[IBIS ver]	1.1
[File name]  	mpc555m.ibs
[File Rev]	0.3
[Date]   Tuesday,04/Dec/2001
[Source]	File originated at Oakhill
[Notes]		Model created by Sukanya Rajagopal(edit rd)
[Disclaimer]	This information is for modeling purposes only
|		and is not guarenteed.
|   This applies to revisions M and later
|   CLKOUT and ECKBUCK output drive changed
|   CLKOUT now 30/90
|   ECKBUCK now 25/50
|   Modified for fast [test] mode vs Normal [slow] comments
|   to agree with reference manual
[Component]	MPC555
[Manufacturer]  Motorola
| Package type  PBGA
[Package]
R_pkg   21.0m   7.00m   36m
L_pkg   3.42nH   0.71nH   6.12nH
C_pkg   0.81pf   0.55pf   1.06pf
[Pin]	  signal_name	model_name	R_pin   L_pin  C_pin
|   mohm   nh   pf
|   POWER AND GROUND PINS
A1	  VDDH		POWER		23	3.81	1.01
A7	  VRL		POWER		25	3.76	0.71
A16	  VDDH		POWER		28	4.13	0.77
A20	  VDDH		POWER		22	3.68	0.97
B2	  VDDH		POWER		23	3.81	1.01
B7	  VRH		POWER		15	2.45	0.72
B19	  VDDH		POWER		22	3.68	0.97
C7	  VDDA		POWER		11	1.77	0.71
D6   VDDI   POWER
D16   VDDI   POWER
D17   VDDL   POWER
E4   VDDL   POWER
J4   VDDSRAM   POWER		8	1.09	0.7
K4   VDDL   POWER
K17   VDDL   POWER
P17   VPP   POWER		19	2.54	0.81
P20   VDDH		POWER   25	3.91	0.72
R17   VDDL   POWER
R18   VDDF		POWER   28	3.9	0.83
R19   XFC		POWER   21	3.06	0.74
R20	  VDDSYN	POWER   27	3.94	0.74
T4   VDDL   POWER
T17   VDDI   POWER
T18	  KAPWR		POWER   19	3.07	0.83
T20	  EXTAL		POWER   27	4.32	0.85
U5   VDDI   POWER
U10   VDDL   POWER
U15   VDDL   POWER
W2	  VDDH		POWER   27	4.11	1.06
W19	  VDDH		POWER   26	4.04	1.03
Y1	  VDDH		POWER   27	4.11	1.06
Y20	  VDDH		POWER   26	4.04	1.03
D7	  VSSA		GND		9	1.27	0.74
P19	  VSSF		GND   15	2.37	0.74
T19	  VSSSYN	GND   22	3.46	0.77
U20	  XTAL		POWER   32	4.76	0.85
|   INPUT ONLY PINS
H3	  CNRX0 	in_5v   26	3.32	0.79
J1	  TCKDXCK	in_3v   23	3.51	0.68
J3	  TRSTB   in_3v   12	1.6	0.69
K1	  TMS		in_3v   23	3.49	0.68
K2	  TDIDSDI	in_3v   17	2.46	0.67
K20	  ACNRX0	in_5v   24	3.58	0.69
M19	  ECK		in_5v   12	2.01	0.71
N17	  RXD1QGP1	in_5v   9	1.29	0.73
N19	  RXD2GP1	in_5v   13	2.12	0.7
P18	  EPEE		in_5v   25	3.34	0.81
U18	  EXTCLK	in_extclk   18	2.93	0.87
V19	  PORESETB	in_3v   30	4.49	0.93
Y18	  IRQ6BMCK2	in_3v   29	4.41	0.8
Y19	  IRQ7BMCK3	in_3v   34	5.14	0.96
|  OUTPUT ONLY PINS
|  Pins in this section have the option of using full strength(50pf load)
|  or half strength(25pf load). The default for these pins use full
|  strength drivers(model : out_3vf). To select half strength drivers
|  (out_3vh), all of the pins in this section must be changed.
|  The models available are:
|  Full strength : out_3vf
|  Half strength : out_3vh
J2	  TDODSDO	out_3vf   18	2.69	0.69
P4	  CS0B		out_3vf   10	1.42	0.73
R2	  CS3B		out_3vf   19	2.96	0.73
R3	  CS2B		out_3vf   26	3.35	0.8
R4	  CS1B		out_3vf   21	3.11	0.81
T1	  OEB		out_3vf   28	4.28	0.75
L1	  IWPIVFLS1	out_3vf   23	3.69	0.69
L2	  IWPOVFLS 	out_3vf   17	2.58	0.68
U17	  RCFBTXP	out_3vf   13	1.89	0.95
|  OUTPUT ONLY PINS
|  Pins in this section have the option of using normal mode or fast [test] mode
|  and the slew rate in both the cases is 200ns.(slow slew rate).The default
|  for these pins operate in normal mode (model : out_5v_200). To select fast
|  [test] mode (out_5v_200tm), all of the pins in this section must be changed.
|  The models available are:
|  Normal mode : out_5v_200
|  fast [test] mode   : out_5v_200tm
H4	  BCNTX0   out_5v_200   17	1.98	0.78
K19	  ACNTX0	out_5v_200   17	2.58	0.69
N18	  TXD1QGP0 	out_5v_200   27	3.59	0.82
N20	  TXD2QGP0 	out_5v_200   20	3.24	0.7
|  OUTPUT ONLY CLOCK PINS
|  5v Eng. clk have the option of using full drive strength(50pf load)
|  or half drive strength(25pf load).The default for this pin uses full
|  strength driver(model : out_5vf_clk). To select half strength driver
|  (out_5vh_clk), the pin in this section must be changed.
|  This pin changed on revision M and later.
|  The models available are:
|  Full Strength : out_5vf_clk
|  Half Strength : out_5vh_clk
U19	  ECKBUCK	out_5vf_clk	 25	3.75	0.84
|  OUTPUT ONLY PINS
|  3v clkout pin have the option of using full drive strength(90pf load)
|  or half drive strength(30pf load).The default for this pin use full
|  strength driver(model : out_3vf_clk). To select half strength driver
|  (out_3vh_clk), the pin in this section must be changed.
|  This pin changed on revision M and later.
|  The models available are:
|  Full Strength : out_3vf_clk
|  Half Strength : out_3vh_clk
V18	  CLKOUT	out_3vf_clk	 23	3.63	0.92
|  I/O PINS(Address & Data) in this section have the option of using 3v
|  driver with full drive strength(50pf load) or half drive strength
|  (25pf load), or 5v driver with 200ns slew rate operating in normal or
|  fast [test] mode. The default is 3v driver with full drive strength
|  (io_35v_3vf).
|  To use other models,all the pins in this section need to be changed.
|  The Pullup and Pulldown data for these models contain both the driver and
|  clamp data. Seperate clamp data is also provided.
|  Available models are:
|   3v buffer with Full Drive strength  : io_35v_3vf
|   3v buffer with Half Drive strength  : io_35v_3vh
|   5v, 200ns slew rate buffer in Normal mode  : io_35v_5v_200
|   5v, 200ns slew rate buffer in fast [test] mode   : io_35v_5v_200tm
V6	  ADDRSGP8	io_35v_3vf   15	2.15	0.79
V5	  ADDRSGP9	io_35v_3vf   16	2.26	0.8
V4	  ADDRSGP10	io_35v_3vf   18	2.64	0.84
V3	  ADDRSGP11	io_35v_3vf   14	2.26	0.85
W1	  ADDRSGP12	io_35v_3vf   33	5.13	0.89
Y2	  ADDRSGP13	io_35v_3vf   33	5.06	0.89
W3	  ADDRSGP14	io_35v_3vf   25	3.8	0.86
Y3	  ADDRSGP15	io_35v_3vf   32	4.78	0.85
W4	  ADDRSGP16	io_35v_3vf   24	3.61	0.84
Y4	  ADDRSGP17	io_35v_3vf   30	4.56	0.82
W5	  ADDRSGP18	io_35v_3vf   21	3.17	0.78
Y5	  ADDRSGP19	io_35v_3vf   28	4.24	0.78
W6	  ADDRSGP20	io_35v_3vf   21	3.07	0.78
Y6	  ADDRSGP21	io_35v_3vf   27	4.08	0.76
V7	  ADDRSGP22	io_35v_3vf   15	2.09	0.75
W7	  ADDRSGP23	io_35v_3vf   20	2.96	0.75
Y7	  ADDRSGP24	io_35v_3vf   27	4.01	0.75
Y8	  ADDRSGP25	io_35v_3vf   26	3.78	0.73
W8	  ADDRSGP26	io_35v_3vf   19	2.81	0.74
V8	  ADDRSGP27	io_35v_3vf   13	1.83	0.74
U8	  ADDRSGP28	io_35v_3vf   8	1.07	0.76
U9	  ADDRSGP29	io_35v_3vf   7	0.82	0.74
U7	  ADDRSGP30	io_35v_3vf   9	1.21	0.78
U6	  ADDRSGP31	io_35v_3vf   8	1.27	0.79
U11	  DATASGP29	io_35v_3vf   7	0.91	0.7
U12	  DATASGP27   io_35v_3vf   8	1.06	0.7
U13	  DATASGP25	io_35v_3vf   9	1.31	0.71
U14	  DATASGP23   io_35v_3vf   9	1.38	0.73
U16	  DATASGP20	io_35v_3vf   13	2.11	0.81
V9	  DATASGP31	io_35v_3vf   13	1.83	0.74
V10	  DATASGP30   io_35v_3vf   12	1.57	0.7
V11	  DATASGP28	io_35v_3vf   11	1.52	0.69
V12	  DATASGP26	io_35v_3vf   11	1.58	0.69
V13	  DATASGP24	io_35v_3vf   12	1.77	0.7
V14	  DATASGP22	io_35v_3vf   12	1.76	0.71
V15   DATASGP21	io_35v_3vf   15	2.25	0.74
V16	  DATASGP19	io_35v_3vf   15	2.28	0.73
V17	  DATASGP18   io_35v_3vf   17	2.61	0.76
W9	  DATASGP1	io_35v_3vf   19	2.77	0.74
W10	  DATASGP3   io_35v_3vf   18	2.58	0.7
W11   DATASGP5   io_35v_3vf   18	2.54	0.7
W12	  DATASGP7	io_35v_3vf   18	2.53	0.69
W13	  DATASGP9   io_35v_3vf   18	2.68	0.71
W14	  DATASGP11   io_35v_3vf   19	2.7	0.72
W15   DATASGP13	io_35v_3vf   19	2.84	0.73
W16	  DATASGP15	io_35v_3vf   20	2.97	0.73
W17	  DATASGP17	io_35v_3vf   21	3.21	0.75
Y9	  DATASGP0	io_35v_3vf   25	3.72	0.72
Y10   DATASGP2	io_35v_3vf   24	3.52	0.69
Y11	  DATASGP4	io_35v_3vf   24	3.51	0.69
Y12	  DATASGP6   io_35v_3vf   24	3.56	0.69
Y13	  DATASGP8	io_35v_3vf   25	3.62	0.71
Y14	  DATASGP10   io_35v_3vf   25	3.69	0.71
Y15	  DATASGP12	io_35v_3vf   26	3.78	0.72
Y16	  DATASGP14	io_35v_3vf   26	3.93	0.74
Y17	  DATASGP16	io_35v_3vf   28	4.1	0.76
|   I/O PINS in this section use 3v supply with 50pf load. To have
|   half the drive strength(25pf load) all the pins in this section
|   need to be changed. Available models are:
|   3v buffer with Full Drive strength  : io_3vf
|   3v buffer with Half Drive strength  : io_3vh
R1	  RDWRB   io_3vf   26	3.84	0.73
T3	  TSIZ1		io_3vf   13	1.97	0.77
U1	  TSIZ0		io_3vf   29	4.55	0.79
U2	  TAB		io_3vf   23	3.33	0.78
U3	  TSB		io_3vf   17	2.75	0.8
U4	  BDIP		io_3vf   14	2.24	0.84
V1	  BURSTB	io_3vf   30	4.62	0.82
V2	  BIBSTSB	io_3vf   20	3.35	0.85
N1	  WEBAT0	io_3vf   24	3.52	0.68
P1	  WEBAT1	io_3vf   26	3.98	0.72
P2	  WEBAT2	io_3vf   20	3.07	0.72
P3	  WEBAT3	io_3vf   13	2.02	0.71
N2	  BRBLWP2	io_3vf   30	3.81	0.77
N3	  BGBLWP1   io_3vf   22	2.8	0.76
N4	  BB_BLWP3	io_3vf   19	2.54	0.78
| I/O PINS in this section use 5v supply with slew rate of 50ns.To have
| fast [test] mode all the pins in this section need to be changed.
| Available modes are:
| 5v fast buffer in normal operation   : io_5v_50
| 5v fast buffer in fast [test] mode operation : io_5v_50tm
L18	  PCS0QGP	io_5v_50   42	5.53	0.91
L17	  PCS1QGP	io_5v_50   41	4.14	0.95
M18	  PCS2QGP	io_5v_50   42	6.12	0.92
M17	  PCS3QGP	io_5v_50   22	2.99	0.87
L19	  MOSIQGP4 	io_5v_50   18	2.51	0.71
L20	  MOSIQGP5	io_5v_50   18	2.96	0.69
M20	  SCKQGP6	io_5v_50   24	3.61	0.69
|   I/O PINS in this section use 5v supply with 200ns slew and
|   operate in normal mode. To operate in fast [test] mode, all the pins
|   in this section need to be changed.
|   Available modes are:
|   5v slow buffer in normal operation   : io_5v_200
|   5v slow buffer in fast [test] mode operation : io_5v_200tm
D3	  ATPUO		io_5v_200   11	1.78	0.94
A2	  ATPU1		io_5v_200   29	4.66	0.96
D4	  ATPU2		io_5v_200   12	1.55	0.64
C3	  ATPU3		io_5v_200   15	2.51	0.86
A3	  ATPU4		io_5v_200   28	4.46	0.85
D5	  ATPU5		io_5v_200   13	1.59	0.64
B3	  ATPU6		io_5v_200   23	3.68	0.87
C4	  ATPU7		io_5v_200   19	2.83	0.84
A4	  ATPU8		io_5v_200   30	4.62	0.83
C5	  ATPU9		io_5v_200   17	2.35	0.72
B4	  ATPU10	io_5v_200   22	3.47	0.79
B5	  ATPU11	io_5v_200   16	2.59	0.74
A5	  ATPU12	io_5v_200   26	3.93	0.73
C6	  ATPU13	io_5v_200   13	1.9	0.6
B6	  ATPU14	io_5v_200   20	2.9	0.74
A6	  ATPU15	io_5v_200   21	3.37	0.71
C2	  AT2CLK	io_5v_200   25	3.85	0.89
H2	  BTPU0		io_5v_200   19	2.69	0.71
H1	  BTPU1		io_5v_200   25	3.83	0.72
G1	  BTPU2		io_5v_200   24	3.67	0.7
G2	  BTPU3		io_5v_200   35	4.65	0.84
G3	  BTPU4		io_5v_200   14	2	0.73
F1	  BTPU5		io_5v_200   26	3.87	0.72
F2	  BTPU6		io_5v_200   36	4.97	0.85
E1	  BTPU7		io_5v_200   29	4.53	0.77
F3	  BTPU8		io_5v_200   14	2.2	0.78
G4	  BTPU9		io_5v_200   10	1.08	0.79
E2	  BTPU10	io_5v_200   22	3.33	0.78
D1	  BTPU11	io_5v_200   28	4.45	0.8
F4	  BTPU12	io_5v_200   21	2.44	0.88
D2	  BTPU13	io_5v_200   22	3.47	0.79
E3	  BTPU14	io_5v_200   19	2.5	0.82
C1	  BTPU15	io_5v_200   30	4.71	0.82
B1	  BT2CLK	io_5v_200   32	5.04	0.86
A17	  MDA4		io_5v_200   25	4.14	0.82
A18	  MDA5		io_5v_200   28	4.51	0.87
A19	  MDA6		io_5v_200   32	5.17	0.94
B17	  MDA7		io_5v_200   20	3.24	0.93
B18	  MDA8		io_5v_200   20	3.35	0.91
C17	  MDA9		io_5v_200   15	2.25	0.94
B20	  MDA10		io_5v_200   31	5	0.93
C18	  MDA11		io_5v_200   20	2.88	0.79
C19	  MDA12		io_5v_200   19	3.07	0.81
C20	  MDA13		io_5v_200   25	4.05	0.8
E17	  MPWM14	io_5v_200   9	1.13	0.78
D18	  MPWM15	io_5v_200   14	2.28	0.77
D19	  MPWM16	io_5v_200   17	2.84	0.77
D20	  MPWM17	io_5v_200   23	3.77	0.76
F17	  MPWM18	io_5v_200   8	0.93	0.76
E18	  MPWM19	io_5v_200   14	2.24	0.76
F18	  MPWM20	io_5v_200   13	1.83	0.75
E19	  MPWM21	io_5v_200   21	3.22	0.75
G17	  MGP105	io_5v_200   7	0.81	0.75
E20	  MGP106	io_5v_200   28	4.33	0.77
F19	  MGP107	io_5v_200   20	2.96	0.74
G18	  MGP108	io_5v_200   13	1.79	0.74
F20	  MGP109	io_5v_200   25	4.01	0.73
H17	  MGP1010	io_5v_200   6	0.8	0.73
G19	  MGP1011	io_5v_200   19	2.86	0.73
G20	  MGP1012	io_5v_200   24	3.81	0.71
H20	  MGP1013	io_5v_200   25	3.83	0.71
H19	  MGP1014	io_5v_200   19	2.81	0.65
H18	  MGP1015	io_5v_200   12	1.78	0.7
J17	  VF2MGP	io_5v_200   6	0.79	0.68
J18	  VFLS0MGP	io_5v_200   11	1.67	0.69
J19	  VF0MGP	io_5v_200   14	2.2	0.69
J20	  VF1MGP	io_5v_200   23	3.45	0.67
K3	  FRZPTR	io_5v_200   11	1.55	0.66
K18	  VFLS1MGP	io_5v_200   7	1.17	0.7
L3	  IRQ3BSGP	io_5v_200   12	1.65	0.68
L4	  IRQ4BSGP	io_5v_200   6	0.71	0.68
M1	  IRQ0BSGP	io_5v_200   23	3.57	0.69
M2	  IRQ1BSGP	io_5v_200   18	2.56	0.68
M3	  IRQ2BSGP	io_5v_200   12	1.89	0.69
M4	  IRQOSGP	io_5v_200   6	0.79	0.67
W18	  IRQ5BSGP	io_5v_200   23	3.52	0.79
| I/O PINS in this section use 3v supply with full strength(25pf) & have
| open_drain structure. To have half strength(50pf load), all the pins
| in this section need to be changed.
| Available models are:
| 3v Open drain buffer with full strength : io_3vf_od
| 3v Open drain buffer with full strength : io_3vf_od
T2	  TEAB		 io_3vf_od   22	3.35	0.76
V20	  SRESETB	 io_3vf_od   33	5.3	0.97
W20	  HRESETB	 io_3vf_od   36	5.65	0.97
| I/O PINS in this section are analog pins which use 5v supply and operate
| in normal mode of operation. To operate in fast [test] mode, these pins
| have to be changed.
| Available models are:
| 5v analog pad in normal mode of opertion : io_5v_an
| 5v analog pad in fast [test] mode of opertion   : io_5v_an_tm
A8	  AAN0PQB0	io_5v_an	20	3.29	0.7
A9	  AAN48PQB4	io_5v_an	19	3.05	0.68
A10	  AAN52PQA0	io_5v_an	19	3.08	0.68
A11	  AAN54PQA2	io_5v_an   25	3.89	0.72
A12	  BAN0PQB0	io_5v_an 	24	3.61	0.7
A13	  BAN2PQB2	io_5v_an	26	3.82	0.72
A14	  BAN3PQB3	io_5v_an	29	4.34	0.78
A15	  BAN51PQB7	io_5v_an	28	4.49	0.78
B8	  AAN3PQB3	io_5v_an	19	2.88	0.7
B9	  AAN49PQB5	io_5v_an	18	2.61	0.69
B10	  AAN53PQA1	io_5v_an 	19	2.67	0.7
B11	  AAN57PQA5	io_5v_an	13	2.17	0.71
B12	  BAN1PQB1	io_5v_an	18	2.64	0.71
B13	  BAN48PQB4	io_5v_an	15	2.45	0.59
B14	  BAN52PQA0	io_5v_an 	21	3.12	0.78
B15	  BAN54PQA2	io_5v_an	21	3.42	0.78
B16	  ETRIG2	io_5v_an	22	3.23	0.78
C8	  AAN2PQB2	io_5v_an	12	1.89	0.71
C9	  AAN51PQB7	io_5v_an	12	1.83	0.7
C10	  AAN56PQA4	io_5v_an	13	1.92	0.74
C11	  AAN59PQA7	io_5v_an   12	1.64	0.7
C12	  BAN49PQB5	io_5v_an	11	1.49	0.55
C13	  BAN53PQA1	io_5v_an	12	1.62	0.58
C14	  BAN56PQA4	io_5v_an	14	1.89	0.79
C15	  BAN57PQA5	io_5v_an	15	2.29	0.67
C16	  ETRIG1	io_5v_an   17	2.49	0.8
D8	  AAN1PQB1	io_5v_an	10	1.38	0.57
D9	  AAN50PQB6	io_5v_an	9	1.23	0.56
D10	  AAN55PQA3	io_5v_an	9	1.15	0.56
D11	  AAN58PQA6	io_5v_an	33	4.19	0.88
D12	  BAN50PQB6	io_5v_an	10	1.14	0.6
D13	  BAN55PQA3	io_5v_an	10	1.14	0.82
D14	  BAN58PQA6	io_5v_an	13	1.53	0.8
D15	  BAN59PQA7	io_5v_an	35	4.28	0.94
| Models and submodels in the file (25): out_3vf (Output), out_3vh (Output), out_5v_200 (Output), out_5v_200tm (Output), out_3vf_clk (Output), out_3vh_clk (Output), out_5vf_clk (Output), out_5vh_clk (Output), io_3vf (I/O), io_3vh (I/O), io_5v_200 (I/O), io_5v_200tm (I/O), io_5v_50 (I/O), io_5v_50tm (I/O), io_35v_3vf (I/O), io_35v_3vh (I/O), io_35v_5v_200 (I/O), io_35v_5v_200tm (I/O), io_3vf_od (I/O), io_3vh_od (I/O), io_5v_an (I/O), io_5v_an_tm (I/O), in_extclk (Input), in_3v (Input), in_5v (Input)
